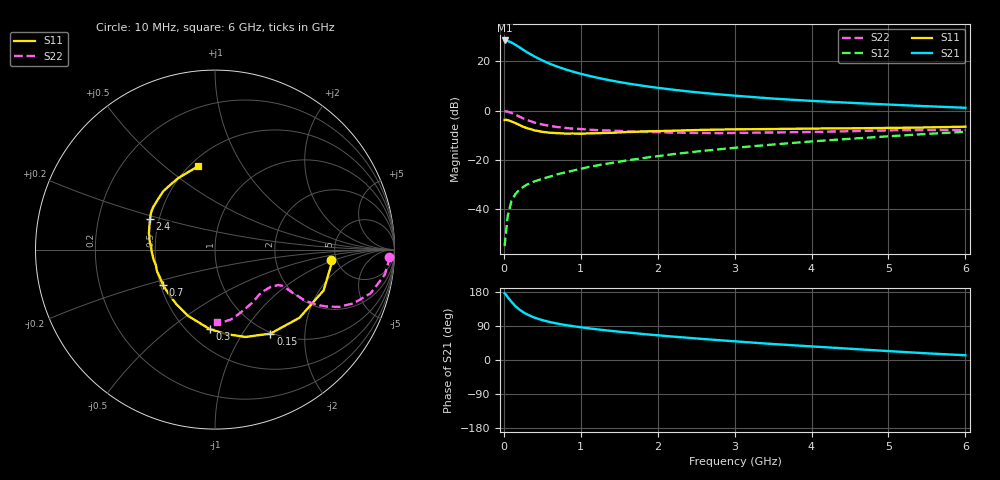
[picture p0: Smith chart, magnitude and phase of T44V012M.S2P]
! Infineon Technologies  Discrete & RF Semiconductors
! BFR182T
! Si NPN RF Bipolar Junction Transistor in SC75
! VCE = 4 V  IC = 12 mA
! Common Emitter S-Parameters:  October  1999
# GHz  S  MA  R  50
!  f  S11  S21  S12  S22
! GHz  MAG  ANG  MAG  ANG  MAG  ANG  MAG  ANG
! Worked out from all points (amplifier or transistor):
!   36 points, 10 MHz to 6 GHz, reference 50 ohm
!   highest |S21| = 28.5 dB at 10 MHz (marker M1)
!   |S21| within 3 dB of that: start of sweep to 214 MHz
!   unconditionally stable (mu >= 1): 907.5 MHz to 3.755 GHz
!   at 250 MHz: K = 0.50, MSG = 27.8 dB, |S12| = -30.9 dB
!   at 1.4 GHz: K = 1.08, MAG = 15.0 dB, |S12| = -21.2 dB
!   at 6 GHz: K = 0.85, MSG = 4.9 dB, |S12| = -8.5 dB
!   S11 on the Smith chart (normalised r, x): 10 MHz: 4.52, -0.94; 150 MHz: 0.98, -1.34; 300 MHz: 0.64, -0.71; 700 MHz: 0.52, -0.23; 2.4 GHz: 0.45, +0.18; 6 GHz: 0.55, +0.66
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0.01  0.6507 -5.3  26.46 176.0  0.0018 75.6  0.9702 -2.4
0.02  0.6543 -6.8  26.24 174.4  0.0026 94.0  0.9716 -3.4
0.05  0.6465 -20.6  25.87 165.8  0.0073 84.1  0.956 -8.4
0.1  0.6045 -39.0  23.99 153.3  0.015 74.5  0.9003 -15.7
0.15  0.5606 -56.6  21.68 142.2  0.0204 68.5  0.8281 -21.2
0.2  0.5157 -70.7  19.37 133.5  0.0249 65.8  0.761 -24.8
0.25  0.4744 -82.7  17.2 126.4  0.0284 61.3  0.6983 -27.0
0.3  0.4438 -93.8  15.35 120.6  0.0319 61.5  0.6498 -28.4
0.4  0.3994 -111.7  12.48 111.6  0.037 60.2  0.5724 -29.6
0.5  0.3728 -125.3  10.43 105.2  0.0417 60.7  0.5251 -29.2
0.6  0.3571 -136.5  8.89 100.1  0.0463 61.1  0.4906 -29.1
0.7  0.3506 -145.5  7.763 95.9  0.0517 63.0  0.4655 -28.7
0.9  0.3452 -159.7  6.156 89.3  0.0611 64.6  0.4323 -28.4
1.1  0.347 -171.0  5.112 83.6  0.0722 65.4  0.4136 -28.9
1.4  0.3563 177.5  4.067 76.7  0.0869 66.9  0.3939 -30.7
1.6  0.3704 170.9  3.584 72.6  0.0983 67.4  0.3817 -31.9
2.2  0.393 157.9  2.661 61.7  0.1315 67.5  0.3616 -38.3
2.4  0.4009 154.4  2.454 58.5  0.1424 67.3  0.3552 -40.8
3.5  0.4248 137.8  1.758 42.1  0.2063 64.0  0.3618 -55.6
4.5  0.4379 125.0  1.444 29.7  0.2696 59.4  0.3841 -70.5
5.5  0.4574 108.8  1.231 17.6  0.3381 53.8  0.4053 -83.2
6  0.4741 101.2  1.145 12.5  0.3741 50.0  0.4054 -88.4
